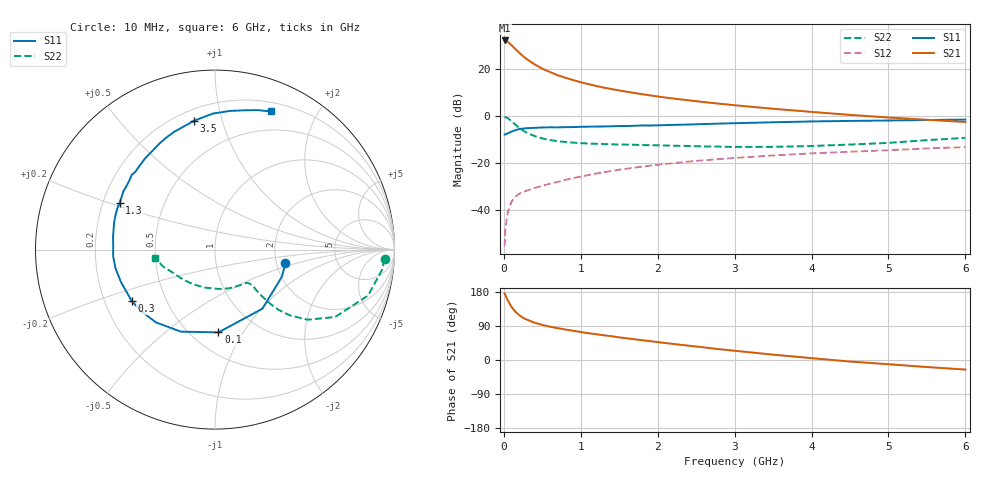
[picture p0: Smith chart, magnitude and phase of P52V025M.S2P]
! SIEMENS Small Signal Semiconductors
! BFP183
! Si NPN RF Bipolar Junction Transistor in SOT143
! VCE = 2 V  IC = 25 mA
! Common Emitter S-Parameters:  March  1996
# GHz  S  MA  R  50
!  f  S11  S21  S12  S22
! GHz  MAG  ANG  MAG  ANG  MAG  ANG  MAG  ANG
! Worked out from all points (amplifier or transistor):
!   36 points, 10 MHz to 6 GHz, reference 50 ohm
!   highest |S21| = 32.0 dB at 10 MHz (marker M1)
!   |S21| within 3 dB of that: start of sweep to 130.8 MHz
!   unconditionally stable (mu >= 1): 627.2 MHz to 5.671 GHz
!   at 250 MHz: K = 0.59, MSG = 28.9 dB, |S12| = -32.5 dB
!   at 1.4 GHz: K = 1.20, MAG = 14.7 dB, |S12| = -23.4 dB
!   at 6 GHz: K = 0.97, MSG = 5.3 dB, |S12| = -13.3 dB
!   S11 on the Smith chart (normalised r, x): 10 MHz: 2.24, -0.40; 100 MHz: 0.67, -0.79; 300 MHz: 0.32, -0.26; 1.3 GHz: 0.27, +0.22; 3.5 GHz: 0.27, +0.82; 6 GHz: 0.29, +1.44
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0.01  0.3993 -10.9  39.77 175.4  0.0017 80.7  0.9465 -3.2
0.02  0.4024 -21.9  39.59 171.1  0.0039 79.1  0.9373 -6.9
0.05  0.4222 -51.2  37.51 157.8  0.0088 75.1  0.8904 -16.7
0.1  0.4616 -87.6  31.6 140.1  0.015 61.0  0.7672 -29.3
0.15  0.4949 -112.5  26.2 127.3  0.0191 54.5  0.6475 -37.1
0.2  0.522 -128.9  21.83 118.2  0.0221 51.0  0.5553 -41.3
0.25  0.5355 -140.0  18.43 111.4  0.0237 49.1  0.4869 -43.5
0.3  0.5451 -148.5  15.9 106.4  0.0258 49.3  0.4345 -44.4
0.4  0.5541 -160.7  12.37 98.4  0.0294 50.0  0.3698 -44.8
0.5  0.5642 -169.5  10.01 92.7  0.0323 50.6  0.3307 -44.6
0.6  0.5688 -176.3  8.49 87.9  0.0363 52.6  0.3052 -44.1
0.7  0.5675 178.1  7.254 83.9  0.0395 53.9  0.2882 -44.0
0.8  0.5726 172.9  6.423 80.3  0.0435 54.9  0.2777 -44.2
1.1  0.5868 160.5  4.699 70.7  0.0552 55.6  0.2572 -46.2
1.3  0.5922 153.8  3.96 65.2  0.0632 55.6  0.251 -48.8
1.7  0.6137 140.8  3.034 54.7  0.0794 54.0  0.2423 -55.4
2.2  0.6402 127.5  2.329 42.4  0.0985 50.4  0.2313 -66.3
2.8  0.6819 113.1  1.805 28.5  0.1203 44.7  0.2213 -82.5
3.5  0.7272 99.2  1.409 14.1  0.1433 38.7  0.2189 -104.6
4.5  0.7773 83.8  1.044 -4.1  0.1722 29.2  0.2448 -137.4
5.5  0.8127 73.0  0.822 -18.6  0.2029 21.1  0.3037 -161.9
6  0.8295 68.1  0.738 -25.2  0.2154 16.4  0.34 -172.4
